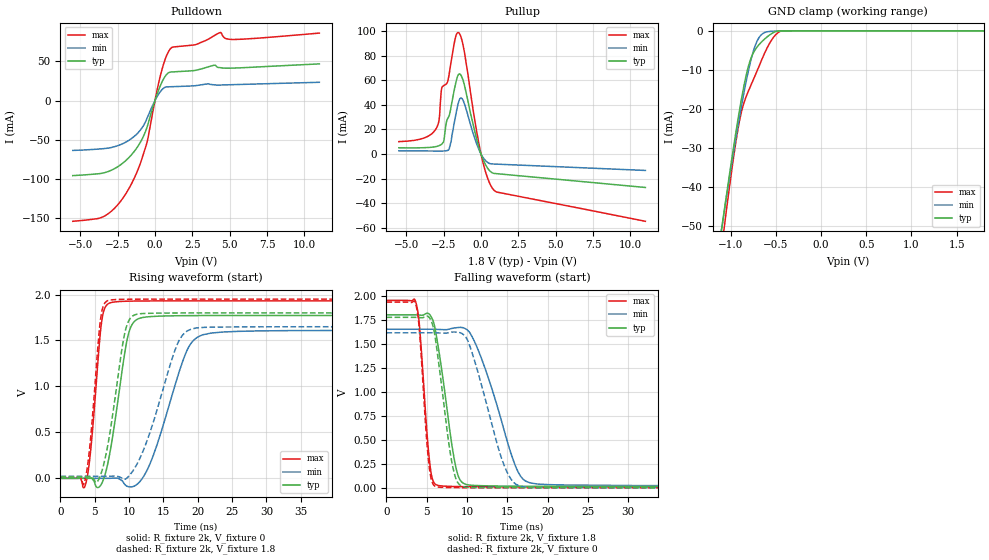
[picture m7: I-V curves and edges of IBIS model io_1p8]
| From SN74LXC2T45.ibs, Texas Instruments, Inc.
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[Model]   io_1p8
Model_type  I/O
Vinl=0.5775
Vinh=1.2675
Enable   Active-Low
Vref =   0
Rref =   2000
Cref =   15p
Vmeas =   0.9
| variable   typ   min   max
C_comp   6.34pF   5.61pF   7.15pF
| C_pullup   10.74pF   6.64pF   16.31pF
| C_pulldown   10.09pF   6.99pF   16.46pF
| C_tri-state   6.34pF   5.61pF   7.15pF
[Temperature Range]   40   100   -40
| Ambient temperature   25   85   -40
[Voltage range]   1.8   1.65   1.95
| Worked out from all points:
|   slope of the pulldown table from 0 to 0.27 V, typ, clamps not added: 18.2 ohm
|   slope of the pullup table from 0 to 0.27 V, typ, clamps not added: 34.2 ohm
|   GND clamp passes 1 mA (typ) near -0.56 V on its own axis
|   rising waveform, R_fixture 2k, V_fixture 0: 20-80 % time 2.1ns typ, 4.01ns min, 1.26ns max; typ from 0 V to 1.77 V
|   falling waveform, R_fixture 2k, V_fixture 1.8: 20-80 % time 1.79ns typ, 3.61ns min, 988ps max; typ from 1.8 V to 0.015 V
|   rising waveform, R_fixture 2k, V_fixture 1.8: 20-80 % time 2.11ns typ, 4.06ns min, 1.25ns max; typ from 0.015 V to 1.8 V
|   falling waveform, R_fixture 2k, V_fixture 0: 20-80 % time 1.65ns typ, 3.18ns min, 935ps max; typ from 1.77 V to 0 V
[GND Clamp]
| LXC8T245_IO_18
|   Voltage   I(typ)   I(min)   I(max)
-5.5V     -897.1mA   -831.9mA   -1.015A
-1.11V    -52.66mA   -52.33mA   -57.72mA
-1.08V    -47.7mA    -47.75mA   -52.14mA
-1.05V    -42.82mA   -43.24mA   -46.67mA
-915mV    -22.23mA   -23.93mA   -24.75mA
-835mV    -12.18mA   -13.81mA   -17.31mA
-785mV    -7.737mA   -8.436mA   -14.47mA
-735mV    -5.102mA   -4.277mA   -11.79mA
-645mV    -2.561mA   -727uA     -6.848mA
-530mV    -501.4uA   -105.7uA   -1.806mA
-430mV    -5.242uA   -35.39uA   -19.91uA
1.8V      23.18pA    30.38nA    510.2pA
[Pulldown]
| LXC8T245_IO_18
|   Voltage   I(typ)   I(min)   I(max)
-5.5V     -95.82mA   -63.67mA   -154.2mA
-3.315V   -91.75mA   -61.14mA   -146.8mA
-1.75V    -72.89mA   -50.79mA   -112.6mA
-1.13V    -58mA      -41.04mA   -87.84mA
-600mV    -37.68mA   -25.69mA   -57.96mA
405mV     21.1mA     12.54mA    35.05mA
770mV     33.15mA    17.47mA    57.09mA
1.105V    36.55mA    17.72mA    67.48mA
2.715V    38.65mA    19.07mA    71.4mA
4.38V     42.01mA    19.88mA    86.86mA
5.235V    41.5mA     20.34mA    78.05mA
11V       46.88mA    23.37mA    86.19mA
[Pullup]
| LXC8T245_IO_18
|   Voltage   I(typ)   I(min)   I(max)
-5.5V     5.088mA    2.627mA    10.09mA
-3.805V   5.165mA    2.515mA    13.04mA
-2.98V    6.16mA     2.455mA    21.15mA
-2.8V     6.846mA    2.441mA    28.18mA
-2.625V   8.108mA    2.443mA    53.57mA
-2.135V   31.01mA    4.02mA     64.57mA
-1.74V    54.87mA    28.55mA    92.96mA
-1.515V   64.43mA    41.57mA    98.64mA
-1.185V   59.29mA    43.25mA    87.57mA
35mV      -1.184mA   -766.3uA   -1.908mA
875mV     -15.72mA   -8.085mA   -29.46mA
11V       -27.14mA   -13.3mA    -54.59mA
[Ramp]
| LXC8T245_IO_18
| variable   typ   min   max
dV/dt_r   1.08/1.1E-09   0.97/1.9E-09   1.159/1.1E-09
dV/dt_f   1.08/1.9E-09   0.99/2E-09   1.17/1.3E-10
R_load = 2k
[Rising Waveform]
| LXC8T245_IO_18
R_fixture =   2k
C_fixture =   0
L_fixture =   0
V_fixture =   0
V_fixture_min = 0
V_fixture_max = 0
|   Time   V(typ)   V(min)   V(max)
0s        267.1pV    9.224nV    2.329nV
3.695ns   -82.43uV   65.71nV    -57.22mV
4.465ns   4.064mV    355.7nV    351.5mV
5.95ns    -65.34mV   -30.39uV   1.675V
7.03ns    209.1mV    -224.7uV   1.903V
9.705ns   1.506V     -86.38mV   1.927V
11.24ns   1.733V     -60.41mV   1.929V
18.23ns   1.77V      1.356V     1.931V
20.03ns   1.771V     1.539V     1.931V
50ns      1.772V     1.61V      1.931V
[Falling Waveform]
| LXC8T245_IO_18
R_fixture =   2k
C_fixture =   0
L_fixture =   0
V_fixture =   1.8
V_fixture_min = 1.65
V_fixture_max = 1.95
|   Time   V(typ)   V(min)   V(max)
0s        1.8V       1.65V      1.95V
3.675ns   1.8V       1.65V      1.922V
4.115ns   1.797V     1.65V      1.669V
5.35ns    1.804V     1.65V      275.4mV
6.2ns     1.582V     1.649V     31.31mV
8.465ns   277.2mV    1.663V     14.23mV
9.7ns     41.09mV    1.66V      12.73mV
16.02ns   17.49mV    227mV      10.6mV
17.4ns    16.87mV    65.62mV    10.44mV
50ns      14.85mV    21.84mV    9.865mV
[Rising Waveform]
| LXC8T245_IO_18
R_fixture =   2k
C_fixture =   0
L_fixture =   0
V_fixture =   1.8
V_fixture_min = 1.65
V_fixture_max = 1.95
|   Time   V(typ)   V(min)   V(max)
0s        14.8mV     21.49mV    9.86mV
3.53ns    14.74mV    21.49mV    -35.27mV
4.34ns    18.83mV    21.49mV    393.9mV
5.795ns   26.31mV    21.47mV    1.706V
6.8ns     322.1mV    21.4mV     1.93V
9.3ns     1.557V     -9.844mV   1.948V
10.73ns   1.776V     101.4mV    1.949V
16.84ns   1.799V     1.427V     1.95V
18.62ns   1.8V       1.61V      1.95V
50ns      1.8V       1.65V      1.95V
[Falling Waveform]
| LXC8T245_IO_18
R_fixture =   2k
C_fixture =   0
L_fixture =   0
V_fixture =   0
V_fixture_min = 0
V_fixture_max = 0
|   Time   V(typ)   V(min)   V(max)
0s        1.774V     1.613V     1.932V
3.64ns    1.774V     1.613V     1.909V
4.08ns    1.771V     1.613V     1.648V
5.25ns    1.778V     1.613V     261mV
6.075ns   1.548V     1.612V     15.29mV
8.09ns    282.1mV    1.62V      2.651mV
9.365ns   16.78mV    1.606V     1.788mV
14.45ns   1.612mV    270mV      731.3uV
16.28ns   1.197mV    28.43mV    562.2uV
50ns      52.81uV    208.2uV    5.463uV
